DATA_BLOCK DB 99
TITLE = Main data block
VERSION : 0.1
STRUCT
	VAR0	: ARRAY  [1 .. 2] OF INT;
	VAR1	: ARRAY  [1 .. 2] OF INT  := 1, 2;
	VAR2	: ARRAY  [1 .. 2, 1 .. 2] OF INT  := 1, 2, 3, 4;
	VAR3	: ARRAY  [-2 .. -1] OF INT := -2, -1;
	VAR4	: ARRAY  [1 .. 2, 1 .. 2, 1 .. 2, 1 .. 2, 1 .. 2, 1 .. 2] OF INT := 4 (1, 2, 3, 4, 5, 6, 7, 8, 9, 10, 11, 12, 13, 14, 15, 16);
	VAR5	: ARRAY  [0 .. 9 ] OF INT := 5 (1, 2);
	VAR6	: ARRAY  [1 .. 2, 1 .. 10, 1 .. 5 ] OF INT := 5 (1, 2, 3, 4, 5, 6, 7, 8, 9, 10, 11, 12, 13, 14, 15, 16, 17, 18, 19, 20);
	VAR7	: ARRAY  [1 .. 14 ] OF BOOL := 7 (TRUE, FALSE);
	VAR8	: ARRAY  [1 .. 3 ] OF BOOL := TRUE, FALSE, TRUE;
	VAR9	: ARRAY  [1 .. 1 ] OF INT := 42;
//	VAR10	: STRUCT
//		VAR10_1		: INT  := 101;
//		VAR10_2		: ARRAY  [1 .. 2 ] OF INT  := 1, 2;
//		VAR10_3		: ARRAY  [1 .. 2 ] OF STRUCT
//			VAR10_3_1	: INT  := 1031;
//			VAR10_3_2	: ARRAY  [1 .. 2 ] OF INT  := 1, 2;
//		END_STRUCT;
//	END_STRUCT;
END_STRUCT;
BEGIN
	VAR0[1]				:= 0;
	VAR0[2]				:= 0;
	VAR1[1]				:= -30000;
	VAR1[2]				:= 30000;
	VAR2[1, 1]			:= 1;
	VAR2[1, 2]			:= 2;
	VAR2[2, 1]			:= 3;
	VAR2[2, 2]			:= 4;
	VAR3[-2]			:= -2;
	VAR3[-1]			:= -1;
	VAR4[1, 1, 1, 1, 1, 1]		:= 1;
	VAR4[1, 1, 1, 1, 1, 2]		:= 2;
	VAR4[1, 1, 1, 1, 2, 1]		:= 3;
	VAR4[1, 1, 1, 1, 2, 2]		:= 4;
	VAR4[1, 1, 1, 2, 1, 1]		:= 5;
	VAR4[1, 1, 1, 2, 1, 2]		:= 6;
	VAR4[1, 1, 1, 2, 2, 1]		:= 7;
	VAR4[1, 1, 1, 2, 2, 2]		:= 8;
	VAR4[1, 1, 2, 1, 1, 1]		:= 9;
	VAR4[1, 1, 2, 1, 1, 2]		:= 10;
	VAR4[1, 1, 2, 1, 2, 1]		:= 11;
	VAR4[1, 1, 2, 1, 2, 2]		:= 12;
	VAR4[1, 1, 2, 2, 1, 1]		:= 13;
	VAR4[1, 1, 2, 2, 1, 2]		:= 14;
	VAR4[1, 1, 2, 2, 2, 1]		:= 15;
	VAR4[1, 1, 2, 2, 2, 2]		:= 16;
	VAR4[1, 2, 1, 1, 1, 1]		:= 1;
	VAR4[1, 2, 1, 1, 1, 2]		:= 2;
	VAR4[1, 2, 1, 1, 2, 1]		:= 3;
	VAR4[1, 2, 1, 1, 2, 2]		:= 4;
	VAR4[1, 2, 1, 2, 1, 1]		:= 5;
	VAR4[1, 2, 1, 2, 1, 2]		:= 6;
	VAR4[1, 2, 1, 2, 2, 1]		:= 7;
	VAR4[1, 2, 1, 2, 2, 2]		:= 8;
	VAR4[1, 2, 2, 1, 1, 1]		:= 9;
	VAR4[1, 2, 2, 1, 1, 2]		:= 10;
	VAR4[1, 2, 2, 1, 2, 1]		:= 11;
	VAR4[1, 2, 2, 1, 2, 2]		:= 12;
	VAR4[1, 2, 2, 2, 1, 1]		:= 13;
	VAR4[1, 2, 2, 2, 1, 2]		:= 14;
	VAR4[1, 2, 2, 2, 2, 1]		:= 15;
	VAR4[1, 2, 2, 2, 2, 2]		:= 16;
	VAR4[2, 1, 1, 1, 1, 1]		:= 1;
	VAR4[2, 1, 1, 1, 1, 2]		:= 2;
	VAR4[2, 1, 1, 1, 2, 1]		:= 3;
	VAR4[2, 1, 1, 1, 2, 2]		:= 4;
	VAR4[2, 1, 1, 2, 1, 1]		:= 5;
	VAR4[2, 1, 1, 2, 1, 2]		:= 6;
	VAR4[2, 1, 1, 2, 2, 1]		:= 7;
	VAR4[2, 1, 1, 2, 2, 2]		:= 8;
	VAR4[2, 1, 2, 1, 1, 1]		:= 9;
	VAR4[2, 1, 2, 1, 1, 2]		:= 10;
	VAR4[2, 1, 2, 1, 2, 1]		:= 11;
	VAR4[2, 1, 2, 1, 2, 2]		:= 12;
	VAR4[2, 1, 2, 2, 1, 1]		:= 13;
	VAR4[2, 1, 2, 2, 1, 2]		:= 14;
	VAR4[2, 1, 2, 2, 2, 1]		:= 15;
	VAR4[2, 1, 2, 2, 2, 2]		:= 16;
	VAR4[2, 2, 1, 1, 1, 1]		:= 1;
	VAR4[2, 2, 1, 1, 1, 2]		:= 2;
	VAR4[2, 2, 1, 1, 2, 1]		:= 3;
	VAR4[2, 2, 1, 1, 2, 2]		:= 4;
	VAR4[2, 2, 1, 2, 1, 1]		:= 5;
	VAR4[2, 2, 1, 2, 1, 2]		:= 6;
	VAR4[2, 2, 1, 2, 2, 1]		:= 7;
	VAR4[2, 2, 1, 2, 2, 2]		:= 8;
	VAR4[2, 2, 2, 1, 1, 1]		:= 9;
	VAR4[2, 2, 2, 1, 1, 2]		:= 10;
	VAR4[2, 2, 2, 1, 2, 1]		:= 11;
	VAR4[2, 2, 2, 1, 2, 2]		:= 12;
	VAR4[2, 2, 2, 2, 1, 1]		:= 13;
	VAR4[2, 2, 2, 2, 1, 2]		:= 14;
	VAR4[2, 2, 2, 2, 2, 1]		:= 15;
	VAR4[2, 2, 2, 2, 2, 2]		:= 16;
	VAR5[0]				:= 1;
	VAR5[1]				:= 2;
	VAR5[2]				:= 1;
	VAR5[3]				:= 2;
	VAR5[4]				:= 1;
	VAR5[5]				:= 2;
	VAR5[6]				:= 1;
	VAR5[7]				:= 2;
	VAR5[8]				:= 1;
	VAR5[9]				:= 2;
	VAR6[1, 1, 1]			:= 1;
	VAR6[1, 1, 2]			:= 2;
	VAR6[1, 1, 3]			:= 3;
	VAR6[1, 1, 4]			:= 4;
	VAR6[1, 1, 5]			:= 5;
	VAR6[1, 2, 1]			:= 6;
	VAR6[1, 2, 2]			:= 7;
	VAR6[1, 2, 3]			:= 8;
	VAR6[1, 2, 4]			:= 9;
	VAR6[1, 2, 5]			:= 10;
	VAR6[1, 3, 1]			:= 11;
	VAR6[1, 3, 2]			:= 12;
	VAR6[1, 3, 3]			:= 13;
	VAR6[1, 3, 4]			:= 14;
	VAR6[1, 3, 5]			:= 15;
	VAR6[1, 4, 1]			:= 16;
	VAR6[1, 4, 2]			:= 17;
	VAR6[1, 4, 3]			:= 18;
	VAR6[1, 4, 4]			:= 19;
	VAR6[1, 4, 5]			:= 20;
	VAR6[1, 5, 1]			:= 1;
	VAR6[1, 5, 2]			:= 2;
	VAR6[1, 5, 3]			:= 3;
	VAR6[1, 5, 4]			:= 4;
	VAR6[1, 5, 5]			:= 5;
	VAR6[1, 6, 1]			:= 6;
	VAR6[1, 6, 2]			:= 7;
	VAR6[1, 6, 3]			:= 8;
	VAR6[1, 6, 4]			:= 9;
	VAR6[1, 6, 5]			:= 10;
	VAR6[1, 7, 1]			:= 11;
	VAR6[1, 7, 2]			:= 12;
	VAR6[1, 7, 3]			:= 13;
	VAR6[1, 7, 4]			:= 14;
	VAR6[1, 7, 5]			:= 15;
	VAR6[1, 8, 1]			:= 16;
	VAR6[1, 8, 2]			:= 17;
	VAR6[1, 8, 3]			:= 18;
	VAR6[1, 8, 4]			:= 19;
	VAR6[1, 8, 5]			:= 20;
	VAR6[1, 9, 1]			:= 1;
	VAR6[1, 9, 2]			:= 2;
	VAR6[1, 9, 3]			:= 3;
	VAR6[1, 9, 4]			:= 4;
	VAR6[1, 9, 5]			:= 5;
	VAR6[1, 10, 1]			:= 6;
	VAR6[1, 10, 2]			:= 7;
	VAR6[1, 10, 3]			:= 8;
	VAR6[1, 10, 4]			:= 9;
	VAR6[1, 10, 5]			:= 10;
	VAR6[2, 1, 1]			:= 11;
	VAR6[2, 1, 2]			:= 12;
	VAR6[2, 1, 3]			:= 13;
	VAR6[2, 1, 4]			:= 14;
	VAR6[2, 1, 5]			:= 15;
	VAR6[2, 2, 1]			:= 16;
	VAR6[2, 2, 2]			:= 17;
	VAR6[2, 2, 3]			:= 18;
	VAR6[2, 2, 4]			:= 19;
	VAR6[2, 2, 5]			:= 20;
	VAR6[2, 3, 1]			:= 1;
	VAR6[2, 3, 2]			:= 2;
	VAR6[2, 3, 3]			:= 3;
	VAR6[2, 3, 4]			:= 4;
	VAR6[2, 3, 5]			:= 5;
	VAR6[2, 4, 1]			:= 6;
	VAR6[2, 4, 2]			:= 7;
	VAR6[2, 4, 3]			:= 8;
	VAR6[2, 4, 4]			:= 9;
	VAR6[2, 4, 5]			:= 10;
	VAR6[2, 5, 1]			:= 11;
	VAR6[2, 5, 2]			:= 12;
	VAR6[2, 5, 3]			:= 13;
	VAR6[2, 5, 4]			:= 14;
	VAR6[2, 5, 5]			:= 15;
	VAR6[2, 6, 1]			:= 16;
	VAR6[2, 6, 2]			:= 17;
	VAR6[2, 6, 3]			:= 18;
	VAR6[2, 6, 4]			:= 19;
	VAR6[2, 6, 5]			:= 20;
	VAR6[2, 7, 1]			:= 1;
	VAR6[2, 7, 2]			:= 2;
	VAR6[2, 7, 3]			:= 3;
	VAR6[2, 7, 4]			:= 4;
	VAR6[2, 7, 5]			:= 5;
	VAR6[2, 8, 1]			:= 6;
	VAR6[2, 8, 2]			:= 7;
	VAR6[2, 8, 3]			:= 8;
	VAR6[2, 8, 4]			:= 9;
	VAR6[2, 8, 5]			:= 10;
	VAR6[2, 9, 1]			:= 11;
	VAR6[2, 9, 2]			:= 12;
	VAR6[2, 9, 3]			:= 13;
	VAR6[2, 9, 4]			:= 14;
	VAR6[2, 9, 5]			:= 15;
	VAR6[2, 10, 1]			:= 16;
	VAR6[2, 10, 2]			:= 17;
	VAR6[2, 10, 3]			:= 18;
	VAR6[2, 10, 4]			:= 19;
	VAR6[2, 10, 5]			:= 20;
	VAR7[1]				:= TRUE;
	VAR7[2]				:= FALSE;
	VAR7[3]				:= TRUE;
	VAR7[4]				:= FALSE;
	VAR7[5]				:= TRUE;
	VAR7[6]				:= FALSE;
	VAR7[7]				:= TRUE;
	VAR7[8]				:= FALSE;
	VAR7[9]				:= TRUE;
	VAR7[10]			:= FALSE;
	VAR7[11]			:= TRUE;
	VAR7[12]			:= FALSE;
	VAR7[13]			:= TRUE;
	VAR7[14]			:= FALSE;
	VAR8[1]				:= TRUE;
	VAR8[2]				:= FALSE;
	VAR8[3]				:= TRUE;
	VAR9[1]				:= 42;
//	VAR10.VAR10_1			:= 101;
//	VAR10.VAR10_2[1]		:= 1;
//	VAR10.VAR10_2[2]		:= 2;
//	VAR10.VAR10_3[1].VAR10_3_1	:= 1031;
//	VAR10.VAR10_3[1].VAR10_3_2[1]	:= 1;
//	VAR10.VAR10_3[1].VAR10_3_2[2]	:= 2;
//	VAR10.VAR10_3[2].VAR10_3_1	:= 1031;
//	VAR10.VAR10_3[2].VAR10_3_2[1]	:= 1;
//	VAR10.VAR10_3[2].VAR10_3_2[2]	:= 2;
END_DATA_BLOCK


FUNCTION FC 1 : VOID
VAR_INPUT
	VAR00	: ARRAY [1 .. 2] OF INT;
	VAR01	: ARRAY [1 .. 2, 0 .. 1] OF INT;
	SELECT	: INT;
END_VAR
VAR_OUTPUT
	VAROUT	: ARRAY [1 .. 2] OF DINT;
END_VAR
BEGIN
	// Only run tests for SELECT=1
	L		#SELECT
	L		1
	<>I
	BEB


	// Check passed parameters
	L		#VAR00[1]
	__ASSERT==	__ACCU 1,	91
	L		#VAR00[2]
	__ASSERT==	__ACCU 1,	92
	L		#VAR01[1, 0]
	__ASSERT==	__ACCU 1,	9100
	L		#VAR01[1, 1]
	__ASSERT==	__ACCU 1,	9101
	L		#VAR01[2, 0]
	__ASSERT==	__ACCU 1,	9102
	L		#VAR01[2, 1]
	__ASSERT==	__ACCU 1,	9103

	L		P##VAR00 // Ptr to array name is ptr to first element
	PUSH
	UD		DW#16#FF000000
	__ASSERT==	__ACCU 1,	DW#16#87000000
	POP
	LAR1
	L		W [AR1, P#0.0]
	__ASSERT==	__ACCU 1,	91


	// Forward FC-parameter to FB
	CALL FB 2, DB 10 (
		VAR0	:= #VAR00,
	)


	// Write the output
	L		L#90001
	T		#VAROUT[1]
	L		L#90002
	T		#VAROUT[2]
END_FUNCTION


FUNCTION_BLOCK FB 1
VAR_INPUT
	VAR0	: ARRAY [1 .. 2] OF INT;
	VAR1	: ARRAY [1 .. 2, 0 .. 1] OF INT;
	VARBOOL	: ARRAY [1 .. 10] OF BOOL;
	SELECT	: INT;
END_VAR
VAR_OUTPUT
	VAROUT	: ARRAY [1 .. 2] OF DINT;
END_VAR
BEGIN
	L		#SELECT
	SPL		ERR
	SPA		M000
	SPA		M001
ERR:	__ASSERT==	1,		2	// Wrong #SELECT


	// Check instance-DB initial values
M000:	L		#VAR0[1]
	__ASSERT==	__ACCU 1,	1
	L		DIW 0
	__ASSERT==	__ACCU 1,	1
	L		#VAR0[2]
	__ASSERT==	__ACCU 1,	2
	L		DIW 2
	__ASSERT==	__ACCU 1,	2
	L		#VAR1[1, 0]
	__ASSERT==	__ACCU 1,	100
	L		DIW 4
	__ASSERT==	__ACCU 1,	100
	L		#VAR1[1, 1]
	__ASSERT==	__ACCU 1,	101
	L		DIW 6
	__ASSERT==	__ACCU 1,	101
	L		#VAR1[2, 0]
	__ASSERT==	__ACCU 1,	102
	L		DIW 8
	__ASSERT==	__ACCU 1,	102
	L		#VAR1[2, 1]
	__ASSERT==	__ACCU 1,	103
	L		DIW 10
	__ASSERT==	__ACCU 1,	103
	U		#VARBOOL[2]
	U		#VARBOOL[3]
	U		#VARBOOL[5]
	U		#VARBOOL[8]
	U		#VARBOOL[9]
	__ASSERT==	__STW VKE,	1
	O		#VARBOOL[1]
	O		#VARBOOL[4]
	O		#VARBOOL[6]
	O		#VARBOOL[7]
	O		#VARBOOL[10]
	__ASSERT==	__STW VKE,	0
	L		DIW 12
	__ASSERT==	__ACCU 1,	W#16#9601

	L		P##VAR0 // Ptr to array name is ptr to first element
	__ASSERT==	__ACCU 1,	DW#16#85000000
	LAR1
	L		W [AR1, P#0.0]
	__ASSERT==	__ACCU 1,	1

	SPA		M500


	// Check passed parameters
M001:	L		#VAR0[1]
	__ASSERT==	__ACCU 1,	91
	L		DIW 0
	__ASSERT==	__ACCU 1,	91
	L		#VAR0[2]
	__ASSERT==	__ACCU 1,	92
	L		DIW 2
	__ASSERT==	__ACCU 1,	92
	L		#VAR1[1, 0]
	__ASSERT==	__ACCU 1,	9100
	L		DIW 4
	__ASSERT==	__ACCU 1,	9100
	L		#VAR1[1, 1]
	__ASSERT==	__ACCU 1,	9101
	L		DIW 6
	__ASSERT==	__ACCU 1,	9101
	L		#VAR1[2, 0]
	__ASSERT==	__ACCU 1,	9102
	L		DIW 8
	__ASSERT==	__ACCU 1,	9102
	L		#VAR1[2, 1]
	__ASSERT==	__ACCU 1,	9103
	L		DIW 10
	__ASSERT==	__ACCU 1,	9103
	U		#VARBOOL[1]
	U		#VARBOOL[4]
	U		#VARBOOL[6]
	U		#VARBOOL[7]
	U		#VARBOOL[10]
	__ASSERT==	__STW VKE,	1
	O		#VARBOOL[2]
	O		#VARBOOL[3]
	O		#VARBOOL[5]
	O		#VARBOOL[8]
	O		#VARBOOL[9]
	__ASSERT==	__STW VKE,	0
	L		DIW 12
	__ASSERT==	__ACCU 1,	W#16#6902

	L		P##VAR0 // Ptr to array name is ptr to first element
	__ASSERT==	__ACCU 1,	DW#16#85000000
	LAR1
	L		W [AR1, P#0.0]
	__ASSERT==	__ACCU 1,	91

	SPA		M500


	// Call FC 1 and forward array parameters
M500:	CALL FC 1 (
		VAR00	:= #VAR0,
		VAR01	:= #VAR1,
		SELECT	:= #SELECT,
		VAROUT	:= #VAROUT,
	)
END_FUNCTION_BLOCK


DATA_BLOCK DB 1
TITLE = FB 1 instance DB
FB 1
BEGIN
	VAR0[1]		:= 1;
	VAR0[2]		:= 2;
	VAR1[1, 0]	:= 100;
	VAR1[1, 1]	:= 101;
	VAR1[2, 0]	:= 102;
	VAR1[2, 1]	:= 103;
	SELECT		:= 0;
	VARBOOL[1]	:= FALSE;
	VARBOOL[2]	:= TRUE;
	VARBOOL[3]	:= TRUE;
	VARBOOL[4]	:= FALSE;
	VARBOOL[5]	:= TRUE;
	VARBOOL[6]	:= FALSE;
	VARBOOL[7]	:= FALSE;
	VARBOOL[8]	:= TRUE;
	VARBOOL[9]	:= TRUE;
	VARBOOL[10]	:= FALSE;
END_DATA_BLOCK


FUNCTION_BLOCK FB 2
VAR_INPUT
	VAR0	: ARRAY [1 .. 2] OF INT;
END_VAR
BEGIN
	L		#VAR0[1]
	__ASSERT==	__ACCU 1,	91
	L		#VAR0[2]
	__ASSERT==	__ACCU 1,	92
END_FUNCTION_BLOCK


DATA_BLOCK DB 10
TITLE = FB 2 instance DB
FB 2
BEGIN
	VAR0[1]		:= 0;
	VAR0[2]		:= 0;
END_DATA_BLOCK


DATA_BLOCK DB 2
TITLE = Parameter passing DB
STRUCT
	VAR0	: ARRAY [1 .. 2] OF INT;
	VAR1	: ARRAY [1 .. 2, 0 .. 1] OF INT;
	VAR2	: ARRAY [1 .. 2] OF DINT;
	VAR3	: ARRAY [1 .. 10] OF BOOL;
END_STRUCT
BEGIN
	VAR0[1]		:= 91;
	VAR0[2]		:= 92;
	VAR1[1, 0]	:= 9100;
	VAR1[1, 1]	:= 9101;
	VAR1[2, 0]	:= 9102;
	VAR1[2, 1]	:= 9103;
	VAR2[1]		:= L#0;
	VAR2[2]		:= L#0;
	VAR3[1]		:= TRUE;
	VAR3[2]		:= FALSE;
	VAR3[3]		:= FALSE;
	VAR3[4]		:= TRUE;
	VAR3[5]		:= FALSE;
	VAR3[6]		:= TRUE;
	VAR3[7]		:= TRUE;
	VAR3[8]		:= FALSE;
	VAR3[9]		:= FALSE;
	VAR3[10]	:= TRUE;
END_DATA_BLOCK


ORGANIZATION_BLOCK OB 1
BEGIN

	// Check DB99 initial values
	L		DB99.VAR0[1]
	__ASSERT==	__ACCU 1,	0
	L		DB99.DBW 0
	__ASSERT==	__ACCU 1,	0
	L		DB99.VAR0[2]
	__ASSERT==	__ACCU 1,	0
	L		DB99.DBW 2
	__ASSERT==	__ACCU 1,	0
	L		DB99.VAR1[1]
	__ASSERT==	__ACCU 1,	-30000
	L		DB99.DBW 4
	__ASSERT==	__ACCU 1,	-30000
	L		DB99.VAR1[2]
	__ASSERT==	__ACCU 1,	30000
	L		DB99.DBW 6
	__ASSERT==	__ACCU 1,	30000
	L		DB99.VAR2[1, 1]
	__ASSERT==	__ACCU 1,	1
	L		DB99.DBW 8
	__ASSERT==	__ACCU 1,	1
	L		DB99.VAR2[1, 2]
	__ASSERT==	__ACCU 1,	2
	L		DB99.DBW 10
	__ASSERT==	__ACCU 1,	2
	L		DB99.VAR2[2, 1]
	__ASSERT==	__ACCU 1,	3
	L		DB99.DBW 12
	__ASSERT==	__ACCU 1,	3
	L		DB99.VAR2[2, 2]
	__ASSERT==	__ACCU 1,	4
	L		DB99.DBW 14
	__ASSERT==	__ACCU 1,	4


	// Call FB 1 without array parameter passing
	CALL FB 1, DB 1 (
		SELECT	:= 0,
	)

	// Call FB 1 with array parameter passing
	L		0
	T		DB2.VAR2[1]
	T		DB2.VAR2[2]
	CALL FB 1, DB 1 (
		VAR0	:= DB2.VAR0,
		VAR1	:= DB2.VAR1,
		VARBOOL	:= DB2.VAR3,
		SELECT	:= 1,
		VAROUT	:= DB2.VAR2,
	)
	L		DB2.VAR2[1]
	__ASSERT==	__ACCU 1,	L#90001
	L		DB2.VAR2[2]
	__ASSERT==	__ACCU 1,	L#90002

	// Call FC 1 with array parameter passing
	L		0
	T		DB2.VAR2[1]
	T		DB2.VAR2[2]
	CALL FC 1 (
		VAR00	:= DB2.VAR0,
		VAR01	:= DB2.VAR1,
		SELECT	:= 1,
		VAROUT	:= DB2.VAR2,
	)
	L		DB2.VAR2[1]
	__ASSERT==	__ACCU 1,	L#90001
	L		DB2.VAR2[2]
	__ASSERT==	__ACCU 1,	L#90002


	CALL SFC 46 // STOP CPU
END_ORGANIZATION_BLOCK
